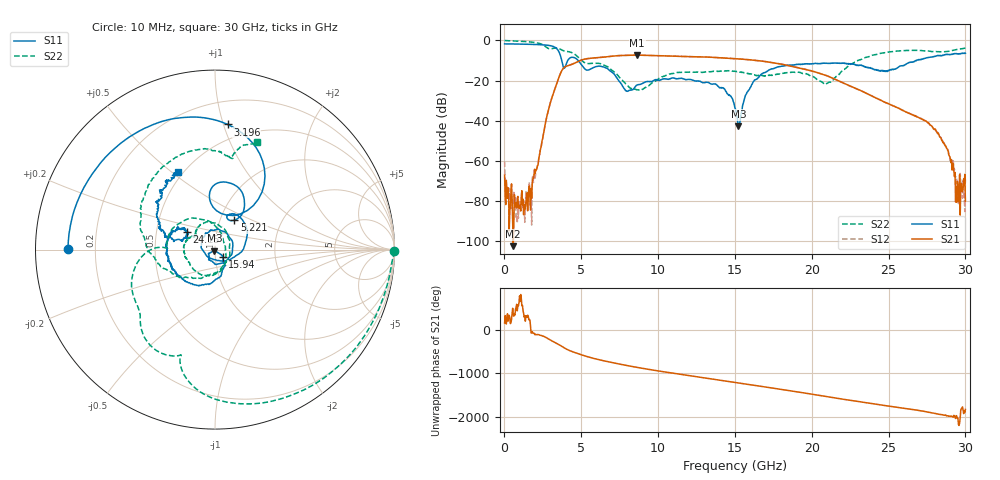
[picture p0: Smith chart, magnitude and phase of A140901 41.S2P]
!  2-Port S-parameters saved by WinCal
! VAR MeasName=S-Parameters (CALIBRATED_DATA) read from VNA (N5244A)
! VAR MeasDate=11/3/2014 9:33:50 AM
! VAR NAME=A140901 41
! VAR FILENAME=A140901 41.S2P
! VAR DATE=11/3/2014 9:33:50 AM
! VAR PHYS_PORTS=1,2
# Hz S RI R 50
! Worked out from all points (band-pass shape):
!   801 points, 10 MHz to 30 GHz, reference 50 ohm
!   highest |S21| = -7.33 dB at 8.632 GHz (marker M1); lowest = -102.5 dB at 572.3 MHz (marker M2)
!   |S21| within 3 dB of the highest: 4.836 GHz to 16.77 GHz (11.94 GHz wide, 110 % of centre)
!   lowest |S11| = -42.7 dB at 15.23 GHz (marker M3), VSWR 1.01, Z = 49.7 - j0.665 ohm
!   |S11| at or under -10 dB: 3.728 GHz to 4.12 GHz (392 MHz wide, 9.99 % of centre); 4.794 GHz to 26.77 GHz (21.98 GHz wide, 139 % of centre); 26.78205 GHz to 26.82375 GHz (41.7 MHz wide, 0.156 % of centre)
!   |S22| runs from -24.7 to 0.0 dB; largest |S21 - S12| = 0.0031
!   S11 on the Smith chart (normalised r, x): 10 MHz: 0.10, +0.00; 3.196 GHz: 0.38, +1.03; 5.221 GHz: 1.17, +0.40; 15.94 GHz: 1.08, -0.09; 24.15 GHz: 0.71, +0.15; 30 GHz: 0.47, +0.53
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1e7  -0.8196 0.00255  -0.000415 0.000149  0.00064 0.00074  0.998 -0.00888
5.723125e8  -0.7942 0.1854  7.44e-06 1.03e-06  9e-05 -1.52e-05  0.904 -0.3512
1.65945e9  -0.6183 0.5061  -8.16e-05 -9.05e-05  -6.24e-05 -6.96e-05  0.432 -0.8088
3.196438e9  0.0698 0.6974  0.00212 0.0499  0.00228 0.0497  -0.2404 -0.5921
4.171112e9  -0.0215 0.3392  -0.0659 -0.2284  -0.0656 -0.2282  -0.4521 -0.2649
5.033325e9  0.1465 0.1911  -0.2638 0.1923  -0.2642 0.192  -0.3154 0.012
5.220762e9  0.1077 0.1644  -0.1834 0.289  -0.184 0.2887  -0.2784 0.01
6.720262e9  0.1796 0.08  0.3864 -0.0778  0.3858 -0.0768  -0.1326 0.1757
8.632125e9  -0.0766 0.00884  -0.3482 -0.2528  -0.348 -0.2527  0.0582 0.0104
1.001916e10  -0.045 0.0917  -0.2905 0.3006  -0.2892 0.3001  0.0427 -0.1006
1.245585e10  0.0979 -0.00168  0.3909 0.0251  0.3901 0.0255  -0.1336 -0.091
1.5005e10  -0.0171 -0.0116  -0.2231 -0.2703  -0.2225 -0.2706  -0.1639 0.0412
1.522992e10  -0.00299 -0.00669  -0.2701 -0.2157  -0.2695 -0.2178  -0.1556 0.0536
1.594219e10  0.0419 -0.0432  -0.3301 -0.00345  -0.3308 -0.0051  -0.126 0.0751
1.755415e10  -0.0536 -0.1927  -0.016 0.2746  -0.0163 0.2749  -0.1082 0.0847
2.002832e10  -0.252 -0.072  0.1252 -0.1181  0.1254 -0.1187  0.0479 0.1172
2.096551e10  -0.2714 -0.0127  -0.0171 -0.1318  -0.0183 -0.1321  0.0823 -0.0151
2.415195e10  -0.1577 0.0993  0.00185 0.037  0.00165 0.0372  -0.4167 0.1505
2.501416e10  -0.1619 0.0645  0.0192 0.0178  0.0191 0.0181  -0.3723 0.3549
2.812562e10  -0.3212 0.2562  -0.00364 -0.00382  -0.00351 -0.00387  0.0768 0.5196
2.947518e10  -0.2571 0.3834  -0.000168 0.000263  -0.000157 7.61e-05  0.153 0.5786
3e10  -0.2079 0.4327  8.19e-05 -5.64e-05  0.000253 -0.00023  0.2338 0.5996
